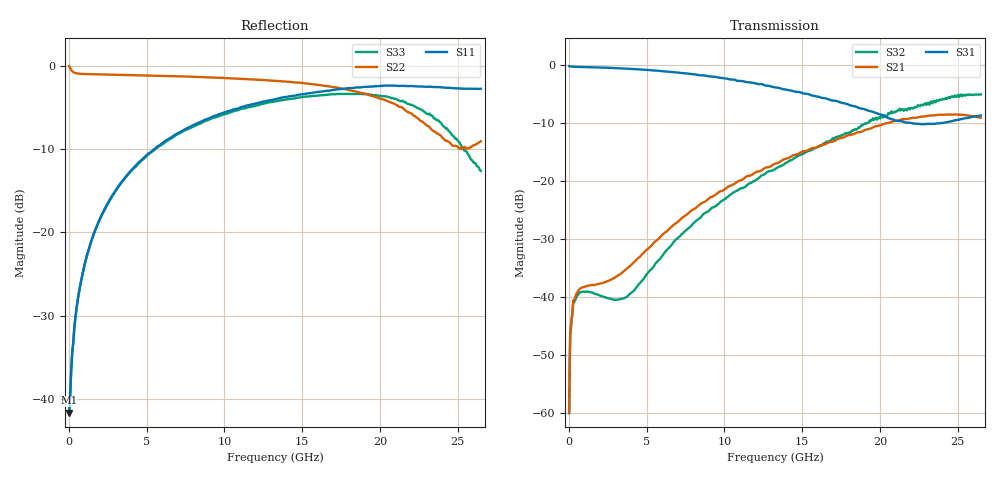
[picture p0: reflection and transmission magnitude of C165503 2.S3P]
!  3-Port S-parameters saved by WinCal
! VAR MeasName=S-Parameters (CALIBRATED_DATA) read from VNA (N5242A)
! VAR MeasDate=2016-5-24 8:49:12
! VAR NAME=C165503 2
! VAR FILENAME=C165503 2.S3P
! VAR DATE=2016-5-24 8:49:12
! VAR PHYS_PORTS=1,2,3
! VAR ObjTypeName=DATASET
! VAR IndexType=Frequency
# Hz S DB R 50
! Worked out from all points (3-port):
!   401 points, 10 MHz to 26.5 GHz, reference 50 ohm
!   strongest paths, dB at 10 MHz, 6.633 GHz, 13.26 GHz, 19.88 GHz, 26.5 GHz:
!     S31: -0.2, -1.2, -3.9, -8.4, -8.7
!     S21: -59.8, -27.8, -17.0, -10.5, -9.1
!     S32: -60.0, -30.9, -18.0, -9.2, -5.1
!   lowest |S11| = -41.7 dB at 10 MHz (marker M1), VSWR 1.02, Z = 50.8 - j0.297 ohm
!   |S11| at or under -10 dB: start of sweep to 5.494 GHz
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1e7  -41.68 -20.7  -59.99 73.5  -0.21 -0.3
     -59.82 43.3  -0.05 -6.1  -57.77 44.7
     -0.20 -0.2  -59.97 59.4  -41.74 -21.2
2.08675e8  -34.51 -97.5  -42.83 43.1  -0.29 -1.7
           -42.87 43.9  -0.66 -94.0  -43.13 40.0
           -0.28 -1.7  -43.09 39.5  -34.45 -99.3
4.0735e8  -30.31 -102.2  -40.03 35.9  -0.32 -2.9
          -39.95 35.9  -0.87 -129.7  -40.34 30.8
          -0.32 -2.9  -40.46 30.6  -30.31 -103.8
1.0696e9  -23.39 -103.0  -38.20 30.0  -0.37 -6.8
          -38.11 30.1  -0.99 -163.0  -38.90 19.1
          -0.37 -6.8  -39.01 19.2  -23.41 -104.7
3.387475e9  -13.96 -111.3  -35.89 64.7  -0.60 -20.8
            -35.83 64.5  -1.09 174.1  -40.14 48.8
            -0.59 -20.7  -40.26 48.9  -14.02 -114.8
5.0431e9  -10.65 -119.5  -31.81 83.8  -0.87 -30.9
          -31.71 83.7  -1.16 165.9  -35.76 81.7
          -0.85 -30.5  -35.89 82.5  -10.76 -124.3
1.3255e10  -4.01 -161.5  -17.10 75.7  -4.00 -75.4
           -16.98 74.8  -1.81 131.2  -17.90 61.5
           -3.87 -75.6  -17.96 62.1  -4.29 -175.5
1.736095e10  -2.83 179.4  -12.74 54.6  -6.51 -92.4
             -12.65 55.1  -2.66 111.6  -12.23 33.5
             -6.36 -92.4  -12.28 32.9  -3.39 157.6
2.106955e10  -2.40 161.8  -10.07 26.8  -9.91 -97.4
             -9.59 30.4  -4.72 92.8  -8.00 -4.2
             -9.57 -97.5  -7.96 -5.5  -4.02 128.7
2.65e10  -2.76 142.3  -9.09 -13.3  -8.75 -94.1
         -9.08 -13.2  -9.07 116.9  -5.10 -70.9
         -8.69 -94.2  -5.06 -71.4  -12.62 116.7
